FUNCTION "GetLEDState" : VOID
TITLE =GetLEDState
//Return status of CPU LED.  LED is selected by LED_Index, which must be one of
//the following values:
// 1: SF (group error)
// 2: INTF (internal error)
// 3: EXTF (external error)
// 4: RUN
// 5: STOP
// 6: FRCE (force)
// 7: CRST (restart)
// 8: BAF (battery fault/overload, short circuit of battery voltage on bus)
// 9: USR (user-defined)
//10: USR1 (user-defined)
//11: BUS1F (bus error interface 1)
//12: BUS2F (bus error interface 2)
//13: REDF (redundancy error)
//14: MSTR (master)
//15: RACK0 (rack number 0)
//16: RACK1 (rack number 1)
//17: RACK2 (rack number 2)
//18: IFM1F (interface error interface module 1)
//19: IFM2F (interface error interface module 2)
VERSION : 0.1


VAR_INPUT
  LED_Index : WORD ;	//LED index from SSL 0x0174
END_VAR
VAR_OUTPUT
  LED_On : BOOL ;	//The specified LED is on
  Flash_Slow : BOOL ;	//true = LED is flashing slowly
  Flash_Fast : BOOL ;	//true = LED is flashing rapidly
END_VAR
VAR_TEMP
  On : BOOL ;	//always on bit
  Busy : BOOL ;
  RVal : INT ;
  NumRec : INT ;
  LED_Int : INT ;	//Led_On as integer
  Flash_Int : INT ;	//LED_Flashing as integer
  SZL_HEADER : STRUCT
   LENTHDR : WORD ;
   N_DR : WORD ;
  END_STRUCT ;
  LED_Data : STRUCT
   CPU : BYTE ;	//F8=Rack0 master, F1=Rack1 stdby, F0=Rack0 Stdby, F9=Rack1 master
   LED_ID : BYTE ;
   LED_ON : BYTE ;	//0=off, 1=on
   LED_Flashing : BYTE ;	//0=none, 1=slow, 2=fast
  END_STRUCT ;
END_VAR
BEGIN
NETWORK
TITLE =Always on bit
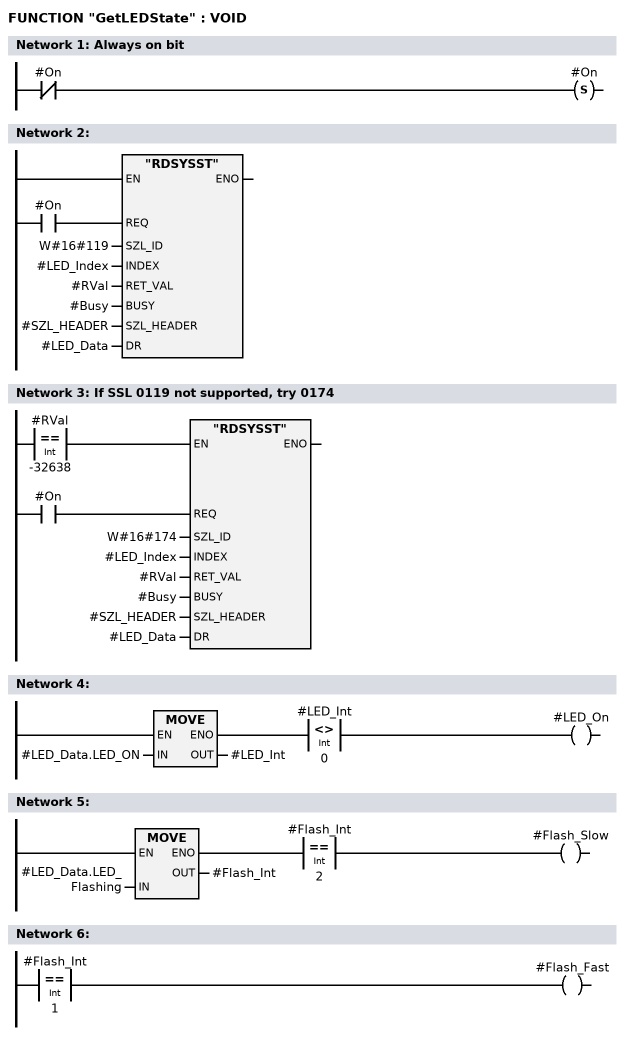
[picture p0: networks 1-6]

      AN    #On;
      S     #On;
NETWORK
TITLE =

      A     #On;
      =     L     18.0;
      BLD   103;
      CALL "RDSYSST" (
           REQ                      := L     18.0,
           SZL_ID                   := W#16#119,
           INDEX                    := #LED_Index,
           RET_VAL                  := #RVal,
           BUSY                     := #Busy,
           SZL_HEADER               := #SZL_HEADER,
           DR                       := #LED_Data);
      NOP   0;
NETWORK
TITLE =If SSL 0119 not supported, try 0174

      A     #On;
      =     L     18.0;
      BLD   103;
      A(    ;
      L     #RVal;
      L     -32638;
      ==I   ;
      )     ;
      JNB   _001;
      CALL "RDSYSST" (
           REQ                      := L     18.0,
           SZL_ID                   := W#16#174,
           INDEX                    := #LED_Index,
           RET_VAL                  := #RVal,
           BUSY                     := #Busy,
           SZL_HEADER               := #SZL_HEADER,
           DR                       := #LED_Data);
_001: NOP   0;
NETWORK
TITLE =

      A(    ;
      L     #LED_Data.LED_ON;
      T     #LED_Int;
      SET   ;
      SAVE  ;
      CLR   ;
      A     BR;
      )     ;
      A(    ;
      L     #LED_Int;
      L     0;
      <>I   ;
      )     ;
      =     #LED_On;
NETWORK
TITLE =

      A(    ;
      L     #LED_Data.LED_Flashing;
      T     #Flash_Int;
      SET   ;
      SAVE  ;
      CLR   ;
      A     BR;
      )     ;
      A(    ;
      L     #Flash_Int;
      L     2;
      ==I   ;
      )     ;
      =     #Flash_Slow;
NETWORK
TITLE =

      L     #Flash_Int;
      L     1;
      ==I   ;
      =     #Flash_Fast;
NETWORK
TITLE =Use ENO to return success/fail state

      A(    ;
      AN    #Busy;
      A(    ;
      L     #RVal;
      L     0;
      ==I   ;
      )     ;
      JNB   _002;
      L     #SZL_HEADER.N_DR;
      T     #NumRec;
      SET   ;
      SAVE  ;
      CLR   ;
_002: A     BR;
      )     ;
      A(    ;
      L     #NumRec;
      L     1;
      ==I   ;
      )     ;
      SAVE  ;
END_FUNCTION

ORGANIZATION_BLOCK OB 1
TITLE = "Main Program Sweep (Cycle)"
VERSION : 0.1


VAR_TEMP
  OB1_EV_CLASS : BYTE ;	//Bits 0-3 = 1 (Coming event), Bits 4-7 = 1 (Event class 1)
  OB1_SCAN_1 : BYTE ;	//1 (Cold restart scan 1 of OB 1), 3 (Scan 2-n of OB 1)
  OB1_PRIORITY : BYTE ;	//Priority of OB Execution
  OB1_OB_NUMBR : BYTE ;	//1 (Organization block 1, OB1)
  OB1_RESERVED_1 : BYTE ;	//Reserved for system
  OB1_RESERVED_2 : BYTE ;	//Reserved for system
  OB1_PREV_CYCLE : INT ;	//Cycle time of previous OB1 scan (milliseconds)
  OB1_MIN_CYCLE : INT ;	//Minimum cycle time of OB1 (milliseconds)
  OB1_MAX_CYCLE : INT ;	//Maximum cycle time of OB1 (milliseconds)
  OB1_DATE_TIME : DATE_AND_TIME ;	//Date and time OB1 started
END_VAR
BEGIN
NETWORK
TITLE =Get state of EXTF LED

      CALL "GetLEDState" (
           LED_Index                := W#16#3,
           LED_On                   := M      0.0,
           Flash_Slow               := M      0.1,
           Flash_Fast               := M      0.2);
      A     BR;
      =     M      0.3;
END_ORGANIZATION_BLOCK

